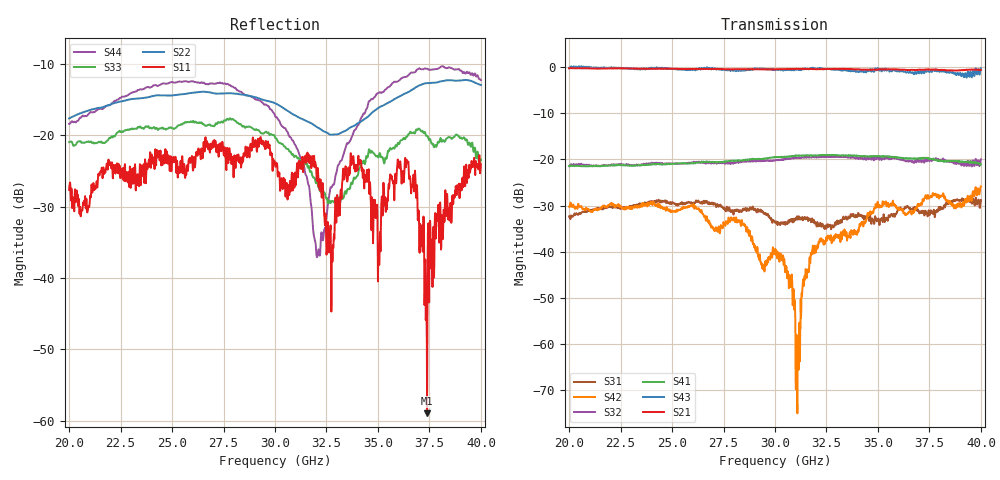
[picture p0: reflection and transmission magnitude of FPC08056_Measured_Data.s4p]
!Keysight Technologies,N5227B,US57180459,A.15.40.08
!Date: Friday, July 21, 2023 10:54:16
!Correction: S11(C  4-Port  )
!S12(C  4-Port  )
!S13(C  4-Port  )
!S14(C  4-Port  )
!S21(C  4-Port  )
!S22(C  4-Port  )
!S23(C  4-Port  )
!S24(C  4-Port  )
!S31(C  4-Port  )
!S32(C  4-Port  )
!S33(C  4-Port  )
!S34(C  4-Port  )
!S41(C  4-Port  )
!S42(C  4-Port  )
!S43(C  4-Port  )
!S44(C  4-Port  )
!S4P File: Measurements: <S11,S12,S13,S14>,
!<S21,S22,S23,S24>,
!<S31,S32,S33,S34>,
!<S41,S42,S43,S44>:
# Hz S  dB  R 50
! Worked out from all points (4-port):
!   1601 points, 20 GHz to 40 GHz, reference 50 ohm
!   strongest paths, dB at 20 GHz, 25 GHz, 30 GHz, 35 GHz, 40 GHz:
!     S21: -0.3, -0.4, -0.5, -0.5, -0.6
!     S43: -0.2, -0.4, -0.7, -0.2, -0.3
!     S41: -21.4, -21.0, -19.5, -19.2, -21.0
!     S32: -21.4, -20.9, -20.3, -19.5, -20.0
!     S42: -30.2, -31.2, -39.5, -29.3, -25.9
!     S31: -32.3, -29.3, -33.7, -33.1, -28.8
!   lowest |S11| = -59.0 dB at 37.39 GHz (marker M1), VSWR 1.00, Z = 49.9 - j0.0502 ohm
!   |S11| at or under -10 dB: start of sweep to end of sweep
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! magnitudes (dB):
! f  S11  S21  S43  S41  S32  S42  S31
! 20 GHz  -27.7  -0.3  -0.2  -21.4  -21.4  -30.2  -32.3
! 28.46 GHz  -23.1  -0.5  -0.8  -20.2  -20.5  -34.1  -30.8
! 31.1 GHz  -25.1  -0.4  -0.5  -19.2  -19.6  -61.1  -33.0
! 32.16 GHz  -26.8  -0.4  -0.3  -19.1  -19.5  -38.0  -34.3
! 36.4 GHz  -23.5  -0.6  -1.2  -19.8  -20.4  -31.9  -30.2
! 37.39 GHz  -59.0  -0.5  -0.9  -19.7  -20.3  -28.4  -31.7
! 40 GHz  -24.1  -0.6  -0.3  -21.0  -20.0  -25.9  -28.8
